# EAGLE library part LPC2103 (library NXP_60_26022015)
Single-chip 16-bit/32-bit microcontrollers; 8 kB/16 kB/32 kB ﬂash with ISP/IAP, fast ports and 10-bit ADC The LPC2101/02/03 microcontrollers are based on a 16-bit/32-bit ARM7TDMI-S CPU with real-time emulation that combines the microcontroller with 8 kB, 16 kB or 32 kB of embedded high-speed ﬂash memory. A 128-bit wide memory interface and a unique accelerator architecture enable 32-bit code execution at the maximum clock rate. For critical performance in interrupt service routines and DSP algorithms, this increases performance up to 30 % over Thumb mode. For critical code size applications, the alternative 16-bit Thumb mode reduces code by more than 30 % with minimal performance penalty. Due to their tiny size and low power consumption, the LPC2101/02/03 are ideal for applications where miniaturization is a key requirement. A blend of serial communications interfaces ranging from multiple UARTs, SPI to SSP and two I2C-buses, combined with on-chip SRAM of 2 kB/4 kB/8 kB, make these devices very well suited for communication gateways and protocol converters. The superior performance also makes these devices suitable for use as math coprocessors. Various 32-bit and 16-bit timers, an improved 10-bit ADC, PWM features through output match on all timers, and 32 fast GPIO lines with up to nine edge or level sensitive external interrupt pins make these microcontrollers particularly suitable for industrial control and medical systems. AAL Eindhoven MK
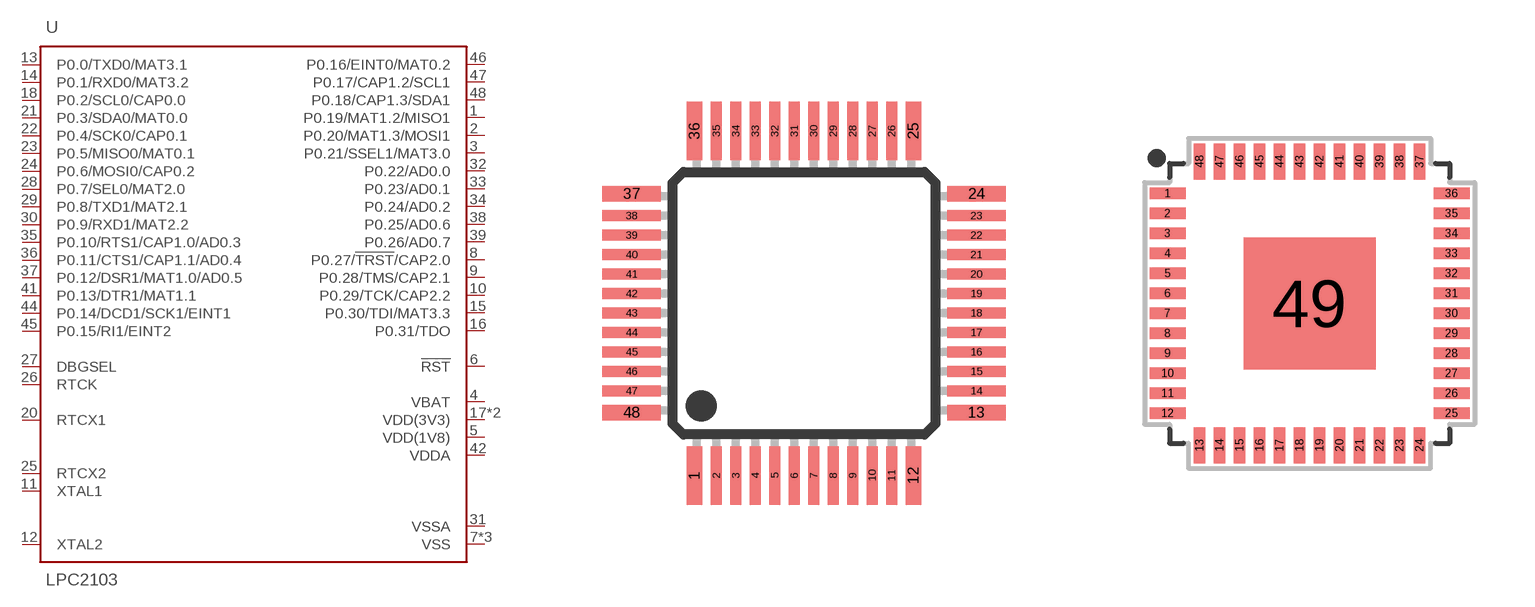
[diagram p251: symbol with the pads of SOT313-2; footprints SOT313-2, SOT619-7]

Designator prefix U

## LPC2103FBD48 (FLASH: 32kB; SRAM: 8kB)  [SOT313-2]
1  P0.19/MAT1.2/MISO1
2  P0.20/MAT1.3/MOSI1
3  P0.21/SSEL1/MAT3.0
4  VBAT  pwr
5  VDD(1V8)  pwr
6  !RST!
7  VSS  pwr
8  P0.27/!TRST!/CAP2.0
9  P0.28/TMS/CAP2.1
10  P0.29/TCK/CAP2.2
11  XTAL1
12  XTAL2
13  P0.0/TXD0/MAT3.1
14  P0.1/RXD0/MAT3.2
15  P0.30/TDI/MAT3.3
16  P0.31/TDO
17  VDD(3V3)  pwr
18  P0.2/SCL0/CAP0.0
19  VSS  pwr
20  RTCX1
21  P0.3/SDA0/MAT0.0
22  P0.4/SCK0/CAP0.1
23  P0.5/MISO0/MAT0.1
24  P0.6/MOSI0/CAP0.2
25  RTCX2
26  RTCK
27  DBGSEL
28  P0.7/SEL0/MAT2.0
29  P0.8/TXD1/MAT2.1
30  P0.9/RXD1/MAT2.2
31  VSSA  pwr
32  P0.22/AD0.0
33  P0.23/AD0.1
34  P0.24/AD0.2
35  P0.10/RTS1/CAP1.0/AD0.3
36  P0.11/CTS1/CAP1.1/AD0.4
37  P0.12/DSR1/MAT1.0/AD0.5
38  P0.25/AD0.6
39  P0.26/AD0.7
40  VDD(3V3)  pwr
41  P0.13/DTR1/MAT1.1
42  VDDA  pwr
43  VSS  pwr
44  P0.14/DCD1/SCK1/EINT1
45  P0.15/RI1/EINT2
46  P0.16/EINT0/MAT0.2
47  P0.17/CAP1.2/SCL1
48  P0.18/CAP1.3/SDA1

## LPC2103FHN48 (FLASH: 32kB; SRAM: 8kB)  [SOT619-7]
Pads as for SOT313-2

## LPC2103FHN48H (FLASH: 32kB; SRAM: 8kB)  [SOT778-3]
Pads as for SOT313-2

## Footprint SOT313-2 (pad centres in mm)
SOT313-2 LQFP48: plastic low profile quad flat package; 48 leads; body 7 x 7 x 1.4 mm JEDEC: MS-026 IEC: 136E05 Footprint according to NXP SOT313-2 specification, however the cornerpins are 0.4mm in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
smd 0.4 x 1.5: 1 -2.81,-4.425; 12 2.81,-4.425; 25 2.81,4.425; 36 -2.81,4.425
smd 0.28 x 1.5: 2 -2.25,-4.425; 3 -1.75,-4.425; 4 -1.25,-4.425; 5 -0.75,-4.425; 6 -0.25,-4.425; 7 0.25,-4.425; 8 0.75,-4.425; 9 1.25,-4.425; 10 1.75,-4.425; 11 2.25,-4.425; 26 2.25,4.425; 27 1.75,4.425; 28 1.25,4.425; 29 0.75,4.425; 30 0.25,4.425; 31 -0.25,4.425; 32 -0.75,4.425; 33 -1.25,4.425; 34 -1.75,4.425; 35 -2.25,4.425
smd 1.5 x 0.4: 13 4.425,-2.81; 24 4.425,2.81; 37 -4.425,2.81; 48 -4.425,-2.81
smd 1.5 x 0.28: 14 4.425,-2.25; 15 4.425,-1.75; 16 4.425,-1.25; 17 4.425,-0.75; 18 4.425,-0.25; 19 4.425,0.25; 20 4.425,0.75; 21 4.425,1.25; 22 4.425,1.75; 23 4.425,2.25; 38 -4.425,2.25; 39 -4.425,1.75; 40 -4.425,1.25; 41 -4.425,0.75; 42 -4.425,0.25; 43 -4.425,-0.25; 44 -4.425,-0.75; 45 -4.425,-1.25; 46 -4.425,-1.75; 47 -4.425,-2.25

## Footprint SOT619-7 (pad centres in mm)
SOT619-7 HVQFN48: plastic thermal enhanced very thin quad flat package; no leads; 48 terminals; body 7 x 7 x 0.85 mm JEDEC: MO-220 IEC: -- JEITA: -- MK
smd 0.9 x 0.29: 1 -3.55,2.75; 2 -3.55,2.25; 3 -3.55,1.75; 4 -3.55,1.25; 5 -3.55,0.75; 6 -3.55,0.25; 7 -3.55,-0.25; 8 -3.55,-0.75; 9 -3.55,-1.25; 10 -3.55,-1.75; 11 -3.55,-2.25; 12 -3.55,-2.75; 25 3.55,-2.75; 26 3.55,-2.25; 27 3.55,-1.75; 28 3.55,-1.25; 29 3.55,-0.75; 30 3.55,-0.25; 31 3.55,0.25; 32 3.55,0.75; 33 3.55,1.25; 34 3.55,1.75; 35 3.55,2.25; 36 3.55,2.75
smd 0.29 x 0.9: 13 -2.75,-3.55; 14 -2.25,-3.55; 15 -1.75,-3.55; 16 -1.25,-3.55; 17 -0.75,-3.55; 18 -0.25,-3.55; 19 0.25,-3.55; 20 0.75,-3.55; 21 1.25,-3.55; 22 1.75,-3.55; 23 2.25,-3.55; 24 2.75,-3.55; 37 2.75,3.55; 38 2.25,3.55; 39 1.75,3.55; 40 1.25,3.55; 41 0.75,3.55; 42 0.25,3.55; 43 -0.25,3.55; 44 -0.75,3.55; 45 -1.25,3.55; 46 -1.75,3.55; 47 -2.25,3.55; 48 -2.75,3.55
smd 3.3 x 3.3: 49 0,0

## Footprint SOT778-3 (pad centres in mm)
SOT778-3 HVQFN48: plastic thermal enhanced very thin quad flat package; no leads; 48 terminals; body 6 x 6 x 0.85 mm JEDEC: -- IEC: -- JEITA: --
smd 0.9 x 0.23: 1 -3.05,2.2; 2 -3.05,1.8; 3 -3.05,1.4; 4 -3.05,1; 5 -3.05,0.6; 6 -3.05,0.2; 7 -3.05,-0.2; 8 -3.05,-0.6; 9 -3.05,-1; 10 -3.05,-1.4; 11 -3.05,-1.8; 12 -3.05,-2.2; 25 3.05,-2.2; 26 3.05,-1.8; 27 3.05,-1.4; 28 3.05,-1; 29 3.05,-0.6; 30 3.05,-0.2; 31 3.05,0.2; 32 3.05,0.6; 33 3.05,1; 34 3.05,1.4; 35 3.05,1.8; 36 3.05,2.2
smd 0.23 x 0.9: 13 -2.2,-3.05; 14 -1.8,-3.05; 15 -1.4,-3.05; 16 -1,-3.05; 17 -0.6,-3.05; 18 -0.2,-3.05; 19 0.2,-3.05; 20 0.6,-3.05; 21 1,-3.05; 22 1.4,-3.05; 23 1.8,-3.05; 24 2.2,-3.05; 37 2.2,3.05; 38 1.8,3.05; 39 1.4,3.05; 40 1,3.05; 41 0.6,3.05; 42 0.2,3.05; 43 -0.2,3.05; 44 -0.6,3.05; 45 -1,3.05; 46 -1.4,3.05; 47 -1.8,3.05; 48 -2.2,3.05
smd 3.8 x 3.8: 49 0,0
